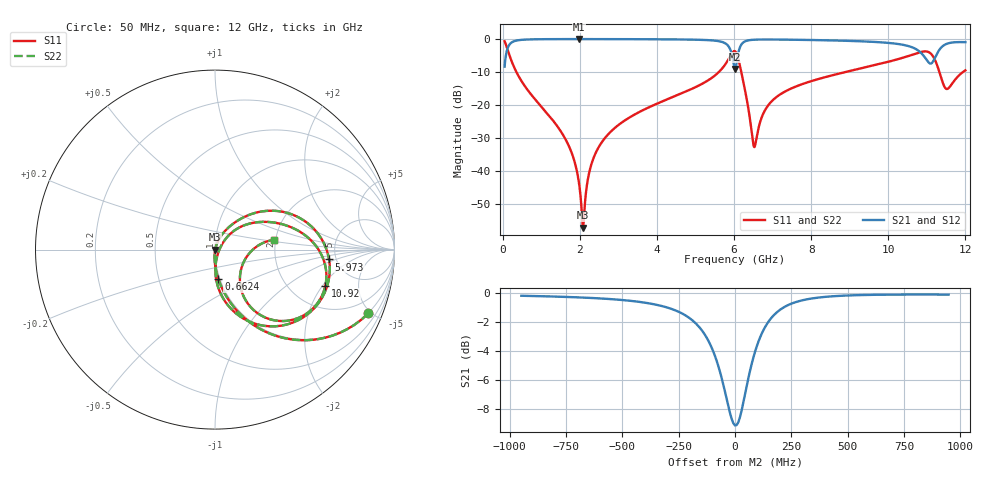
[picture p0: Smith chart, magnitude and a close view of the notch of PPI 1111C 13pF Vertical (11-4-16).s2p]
# GHz S MA R 50
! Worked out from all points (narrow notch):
!   1601 points, 50 MHz to 12 GHz, reference 50 ohm
!   highest |S21| = -0.01 dB at 1.977 GHz (marker M1); lowest = -9.1 dB at 6.025 GHz (marker M2)
!   notch at M2: 8.9 dB deep, 159 MHz wide at half that depth
!   lowest |S11| = -57.3 dB at 2.082 GHz (marker M3), VSWR 1.00, Z = 50.1 - j0.0382 ohm
!   |S11| at or under -10 dB: 354.9 MHz to 5.608 GHz (5.253 GHz wide, 176 % of centre); 6.188 GHz to 8.898 GHz (2.709 GHz wide, 35.9 % of centre); 11.33 GHz to 11.94 GHz (614.3 MHz wide, 5.28 % of centre)
!   |S22| runs from -57.3 to -0.7 dB; largest |S21 - S12| = 0
!   S11 on the Smith chart (normalised r, x): 50 MHz: 0.98, -4.82; 662.4 MHz: 0.98, -0.33; 5.973 GHz: 4.37, -0.80; 10.92 GHz: 3.08, -2.13; 12 GHz: 1.97, +0.24
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0.05  0.9249 -22.6  0.3802 67.4  0.3802 67.4  0.9249 -22.6
0.259125  0.4198 -66.4  0.9071 23.6  0.9071 23.6  0.4198 -66.4
0.6624375  0.1638 -83.5  0.9857 6.2  0.9857 6.2  0.1638 -83.5
1.625906  0.03034 -93.9  0.9982 -6.1  0.9982 -6.1  0.03034 -93.9
1.976938  0.006625 -87.7  0.9985 -9.2  0.9985 -9.2  0.006625 -87.7
2.044156  0.002736 -70.3  0.9985 -9.8  0.9985 -9.8  0.002736 -70.3
2.0815  0.001364 -16.2  0.9985 -10.1  0.9985 -10.1  0.001364 -16.2
2.283156  0.01155 71.2  0.9984 -11.7  0.9984 -11.7  0.01155 71.2
2.566969  0.02689 72.8  0.998 -13.9  0.998 -13.9  0.02689 72.8
4.038312  0.1065 63.3  0.9917 -25.5  0.9917 -25.5  0.1065 63.3
5.472313  0.27 45.6  0.9497 -41.6  0.9497 -41.6  0.27 45.6
5.972719  0.6378 -4.9  0.485 -59.6  0.485 -59.6  0.6378 -4.9
6.025  0.6533 -24.7  0.3505 -35.6  0.3505 -35.6  0.6533 -24.7
6.211719  0.272 -80.8  0.8569 -15.0  0.8569 -15.0  0.272 -80.8
6.525406  0.02283 -20.7  0.9771 -31.0  0.9771 -31.0  0.02283 -20.7
6.966062  0.1119 46.1  0.9839 -39.1  0.9839 -39.1  0.1119 46.1
8.019156  0.2309 37.9  0.9666 -50.6  0.9666 -50.6  0.2309 37.9
10.01331  0.4535 15.1  0.8728 -72.6  0.8728 -72.6  0.4535 15.1
10.91703  0.647 -18.1  0.5571 -86.1  0.5571 -86.1  0.647 -18.1
11.17844  0.5244 -49.0  0.4752 -51.6  0.4752 -51.6  0.5244 -49.0
11.50706  0.1748 -27.8  0.8423 -56.3  0.8423 -56.3  0.1748 -27.8
12  0.3345 9.4  0.8973 -72.8  0.8973 -72.8  0.3345 9.4
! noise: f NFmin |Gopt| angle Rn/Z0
0.05  0.0003835  0.8732  1.564  0.0006519
1.372  0.003817  0.6786  6.876  0.002287
2.701  0.006429  0.6365  12.83  0.003293
4.031  0.009529  0.6385  18.69  0.004848
5.36  0.02181  0.7763  25  0.01903
6.682  0.02995  0.7985  31.34  0.02856
8.012  0.0208  0.6832  36.23  0.01154
9.341  0.02776  0.7248  41.66  0.01756
10.67  0.09951  0.9058  48.03  0.1934
12  0.06904  0.8559  53.19  0.08199
